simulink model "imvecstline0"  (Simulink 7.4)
settings: Solver=ode45  StartTime=0.0  StopTime=2.5  MaxStep=5e-4  RelTol=1e-3

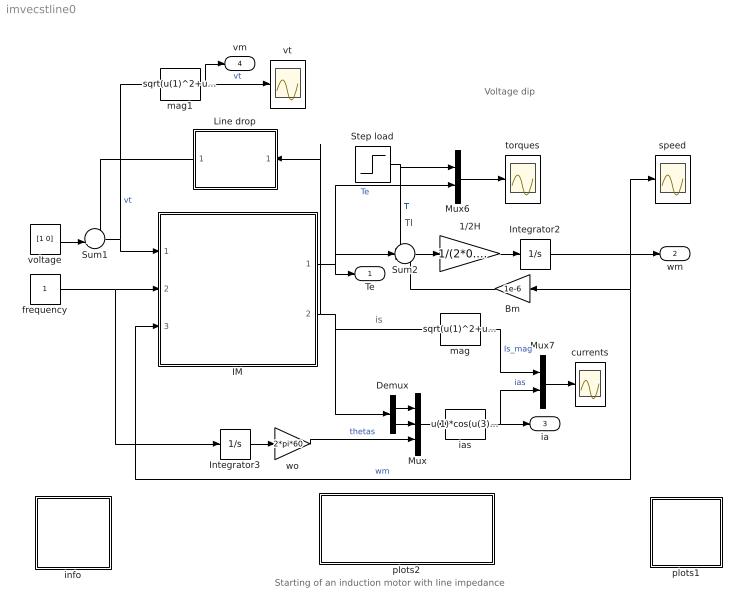
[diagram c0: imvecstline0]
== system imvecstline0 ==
  note: is
  note: Starting of an induction motor with line impedance
  note: Voltage dip
  note: Tl
  1/2H : Gain  Gain=1/(2*0.3)  ParameterDataType=sfix(16)  ParameterScaling=2^0  OutDataType=sfix(16)  OutScaling=2^0
  Bm : Gain  Gain=1e-6  ParameterDataType=sfix(16)  ParameterScaling=2^0  OutDataType=sfix(16)  OutScaling=2^0
  Demux : Demux  Outputs=2
  IM : Subsystem  mask(Inductionmachine){Rs=0.01, Rr=0.02, Lsl=0.10, Lrl=0.10, Lm=4.50, wo=2*pi*60}
      mask prompts: Rs "Stator resistance [pu]"; Rr "Rotor resistance [pu]"; Lsl "Stator leakage inductance [pu]"; Lrl "Rotor leakage inductance [pu]"; Lm "Magnetizing inductance [pu]"; wo "Base frequency [rad/s]"
      mask help: Induction motor subsystem model using state space formulation in an arbitrary reference frame k. Parameters are expressed in per unit.
  Integrator2 : Integrator
  Integrator3 : Integrator
  Line drop : Subsystem  mask{Rline=0.01, Lline=0.05, wo=2*pi*60}
      mask prompts: Rline "Rline [ pu]"; Lline "Lline [pu]"; wo "wo [rad/s]"
  Mux : Mux  Inputs=3
  Mux6 : Mux  Inputs=2
  Mux7 : Mux  Inputs=2
  Step load : Step  Time=2  Before=0.0  SampleTime=0
  Sum1 : Sum  Inputs=-+|  OutDataType=sfix(16)  OutScaling=2^0
  Sum2 : Sum  Inputs=-+-  OutDataType=sfix(16)  OutScaling=2^0
  currents : Scope
  frequency : Constant  OutDataType=sfix(16)  OutScaling=2^0
  ias : Fcn  Expr=u(1)*cos(u(3))-u(2)*sin(u(3))
  info : Subsystem
  mag : Fcn  Expr=sqrt(u(1)^2+u(2)^2)
  mag1 : Fcn  Expr=sqrt(u(1)^2+u(2)^2)
  plots1 : Subsystem
  plots2 : Subsystem
  speed : Scope
  torques : Scope
  voltage : Constant  Value=[1 0]  OutDataType=sfix(16)  OutScaling=2^0
  vt : Scope
  wo : Gain  Gain=2*pi*60  ParameterDataType=sfix(16)  ParameterScaling=2^0  OutDataType=sfix(16)  OutScaling=2^0
  Te : Outport
  wm : Outport  Port=2
  ia : Outport  Port=3
  vm : Outport  Port=4
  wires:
  frequency/1 -> Integrator3/1, IM/2(wk)
  Demux/1 -> Mux/1
  Demux/2 -> Mux/2
  mag/1 -> Mux7/1  "Is_mag"
  Sum2/1 -> 1/2H/1
  1/2H/1 -> Integrator2/1
  wo/1 -> Mux/3  "thetas"
  Bm/1 -> Sum2/3
  Integrator2/1 -> IM/3(wm), Bm/1, speed/1, wm/1  "wm"
  IM/1(Te) -> Sum2/2, Mux6/2, Te/1  "Te"
  IM/2(is) -> mag/1, Demux/1, Line drop/1(i_in)
  Mux6/1 -> torques/1
  Step load/1 -> Mux6/1, Sum2/1  "Tl"
  voltage/1 -> Sum1/2
  Line drop/1(v_out) -> Sum1/1
  Mux/1 -> ias/1
  Integrator3/1 -> wo/1
  Sum1/1 -> IM/1(vs), mag1/1  "vt"
  mag1/1 -> vt/1, vm/1  "vt"
  Mux7/1 -> currents/1
  ias/1 -> Mux7/2, ia/1  "ias"

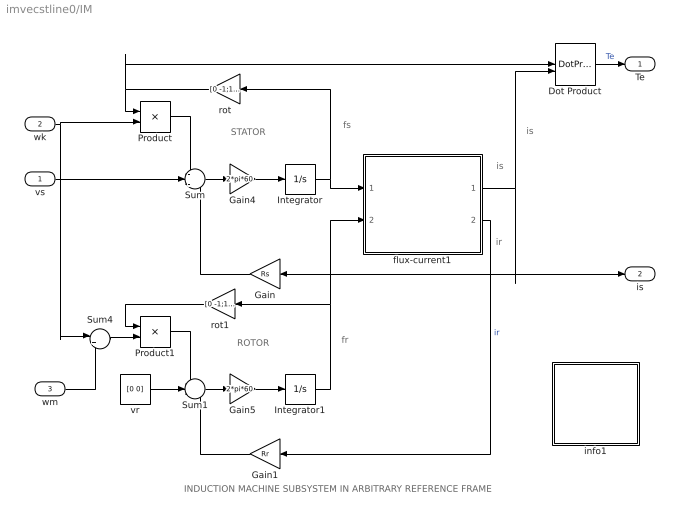
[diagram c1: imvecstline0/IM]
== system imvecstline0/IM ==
  note: ROTOR
  note: STATOR
  note: fs
  note: fr
  note: is
  note: is
  note: INDUCTION MACHINE SUBSYSTEM IN ARBITRARY REFERENCE FRAME
  note: ir
  vs : Inport  OutDataType=sfix(16)  OutScaling=2^0
  wk : Inport  Port=2  OutDataType=sfix(16)  OutScaling=2^0
  wm : Inport  Port=3  OutDataType=sfix(16)  OutScaling=2^0
  Dot Product : DotProduct  OutDataType=fixdt(1, 16)  OutScaling=2^-10
  Gain : Gain  Gain=Rs  ParameterDataType=sfix(16)  ParameterScaling=2^0  OutDataType=sfix(16)  OutScaling=2^0
  Gain1 : Gain  Gain=Rr  ParameterDataType=sfix(16)  ParameterScaling=2^0  OutDataType=sfix(16)  OutScaling=2^0
  Gain4 : Gain  Gain=2*pi*60  ParameterDataType=sfix(16)  ParameterScaling=2^0  OutDataType=sfix(16)  OutScaling=2^0
  Gain5 : Gain  Gain=2*pi*60  ParameterDataType=sfix(16)  ParameterScaling=2^0  OutDataType=sfix(16)  OutScaling=2^0
  Integrator : Integrator  InitialCondition=[0 0]
  Integrator1 : Integrator  InitialCondition=[0 0]
  Product : Product  OutDataType=sfix(16)  OutScaling=2^0
  Product1 : Product  OutDataType=sfix(16)  OutScaling=2^0
  Sum : Sum  Inputs=-+-  OutDataType=sfix(16)  OutScaling=2^0
  Sum1 : Sum  Inputs=-+-  OutDataType=sfix(16)  OutScaling=2^0
  Sum4 : Sum  Inputs=|+-  OutDataType=sfix(16)  OutScaling=2^0
  flux-current1 : Subsystem
  info1 : Subsystem
  rot : Gain  Gain=[0 -1;1 0]  Multiplication=Matrix(K*u)  ParameterDataType=sfix(16)  ParameterScaling=2^0  OutDataType=sfix(16)  OutScaling=2^0
  rot1 : Gain  Gain=[0 -1;1 0]  Multiplication=Matrix(K*u)  ParameterDataType=sfix(16)  ParameterScaling=2^0  OutDataType=sfix(16)  OutScaling=2^0
  vr : Constant  Value=[0 0]  OutDataType=sfix(16)  OutScaling=2^0
  Te : Outport
  is : Outport  Port=2
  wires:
  Gain/1 -> Sum/3
  vr/1 -> Sum1/2
  Gain1/1 -> Sum1/3
  flux-current1/2(ir) -> Gain1/1  "ir"
  Integrator/1 -> flux-current1/1(fs), rot/1
  Integrator1/1 -> flux-current1/2(fr), rot1/1
  Product1/1 -> Sum1/1
  rot1/1 -> Product1/1
  Product/1 -> Sum/1
  rot/1 -> Product/1, Dot Product/1
  Sum4/1 -> Product1/2
  Sum/1 -> Gain4/1
  Gain4/1 -> Integrator/1
  Sum1/1 -> Gain5/1
  Gain5/1 -> Integrator1/1
  flux-current1/1(is) -> Gain/1, is/1, Dot Product/2
  Dot Product/1 -> Te/1  "Te"
  vs/1 -> Sum/2
  wk/1 -> Product/2, Sum4/1
  wm/1 -> Sum4/2

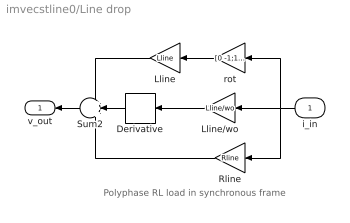
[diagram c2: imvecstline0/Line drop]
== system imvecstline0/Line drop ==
  note: Polyphase RL load in synchronous frame
  i_in : Inport  OutDataType=sfix(16)  OutScaling=2^0
  Derivative : Derivative
  Lline : Gain  Gain=Lline  ParameterDataType=sfix(16)  ParameterScaling=2^0  OutDataType=sfix(16)  OutScaling=2^0
  Lline/wo : Gain  Gain=Lline/wo  ParameterDataType=sfix(16)  ParameterScaling=2^0  OutDataType=sfix(16)  OutScaling=2^0
  Rline : Gain  Gain=Rline  ParameterDataType=sfix(16)  ParameterScaling=2^0  OutDataType=sfix(16)  OutScaling=2^0
  Sum2 : Sum  Inputs=+++  OutDataType=sfix(16)  OutScaling=2^0
  rot : Gain  Gain=[0 -1;1 0]  Multiplication=Matrix(K*u)  ParameterDataType=sfix(16)  ParameterScaling=2^0  OutDataType=sfix(16)  OutScaling=2^0
  v_out : Outport
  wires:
  Sum2/1 -> v_out/1
  Lline/wo/1 -> Derivative/1
  i_in/1 -> Lline/wo/1, rot/1, Rline/1
  rot/1 -> Lline/1
  Derivative/1 -> Sum2/2
  Lline/1 -> Sum2/1
  Rline/1 -> Sum2/3

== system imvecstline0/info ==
  note: Starting of an induction motor
  note: This demonstration illustrates the line starting of an induction motor at no load in the presence of a line impedance between the source and the motor.You will be able to observe the voltage dip associated with the high initial inrush current. To modify the machine parameters, double click the induction motor block.

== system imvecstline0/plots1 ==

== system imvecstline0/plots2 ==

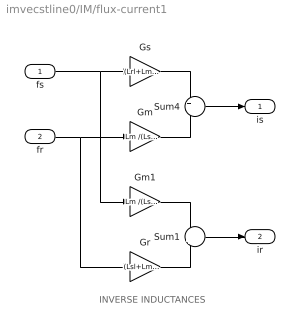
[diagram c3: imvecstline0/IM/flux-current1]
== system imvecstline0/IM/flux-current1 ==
  note: INVERSE INDUCTANCES
  fs : Inport  OutDataType=sfix(16)  OutScaling=2^0
  fr : Inport  Port=2  OutDataType=sfix(16)  OutScaling=2^0
  Gm : Gain  Gain=Lm /(Lsl*Lrl+Lsl*Lm+Lrl*Lm)  ParameterDataType=sfix(16)  ParameterScaling=2^0  OutDataType=sfix(16)  OutScaling=2^0
  Gm1 : Gain  Gain=Lm /(Lsl*Lrl+Lsl*Lm+Lrl*Lm)  ParameterDataType=sfix(16)  ParameterScaling=2^0  OutDataType=sfix(16)  OutScaling=2^0
  Gr : Gain  Gain=(Lsl+Lm )/(Lsl*Lrl+Lsl*Lm+Lrl*Lm)  ParameterDataType=sfix(16)  ParameterScaling=2^0  OutDataType=sfix(16)  OutScaling=2^0
  Gs : Gain  Gain=(Lrl+Lm) /(Lsl*Lrl+Lsl*Lm+Lrl*Lm)  ParameterDataType=sfix(16)  ParameterScaling=2^0  OutDataType=sfix(16)  OutScaling=2^0
  Sum1 : Sum  Inputs=-+  OutDataType=sfix(16)  OutScaling=2^0
  Sum4 : Sum  Inputs=+-  OutDataType=sfix(16)  OutScaling=2^0
  is : Outport
  ir : Outport  Port=2
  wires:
  fs/1 -> Gs/1, Gm1/1
  Gs/1 -> Sum4/1
  fr/1 -> Gm/1, Gr/1
  Gm/1 -> Sum4/2
  Sum4/1 -> is/1
  Gm1/1 -> Sum1/1
  Gr/1 -> Sum1/2
  Sum1/1 -> ir/1

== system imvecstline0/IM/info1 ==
  note: This demonstration illustrates the dynamics of a synchronous generator, initially at no load, following a three-phase short circuit at the terminals.
  note: Synchronous machine transients under shortcircuit
